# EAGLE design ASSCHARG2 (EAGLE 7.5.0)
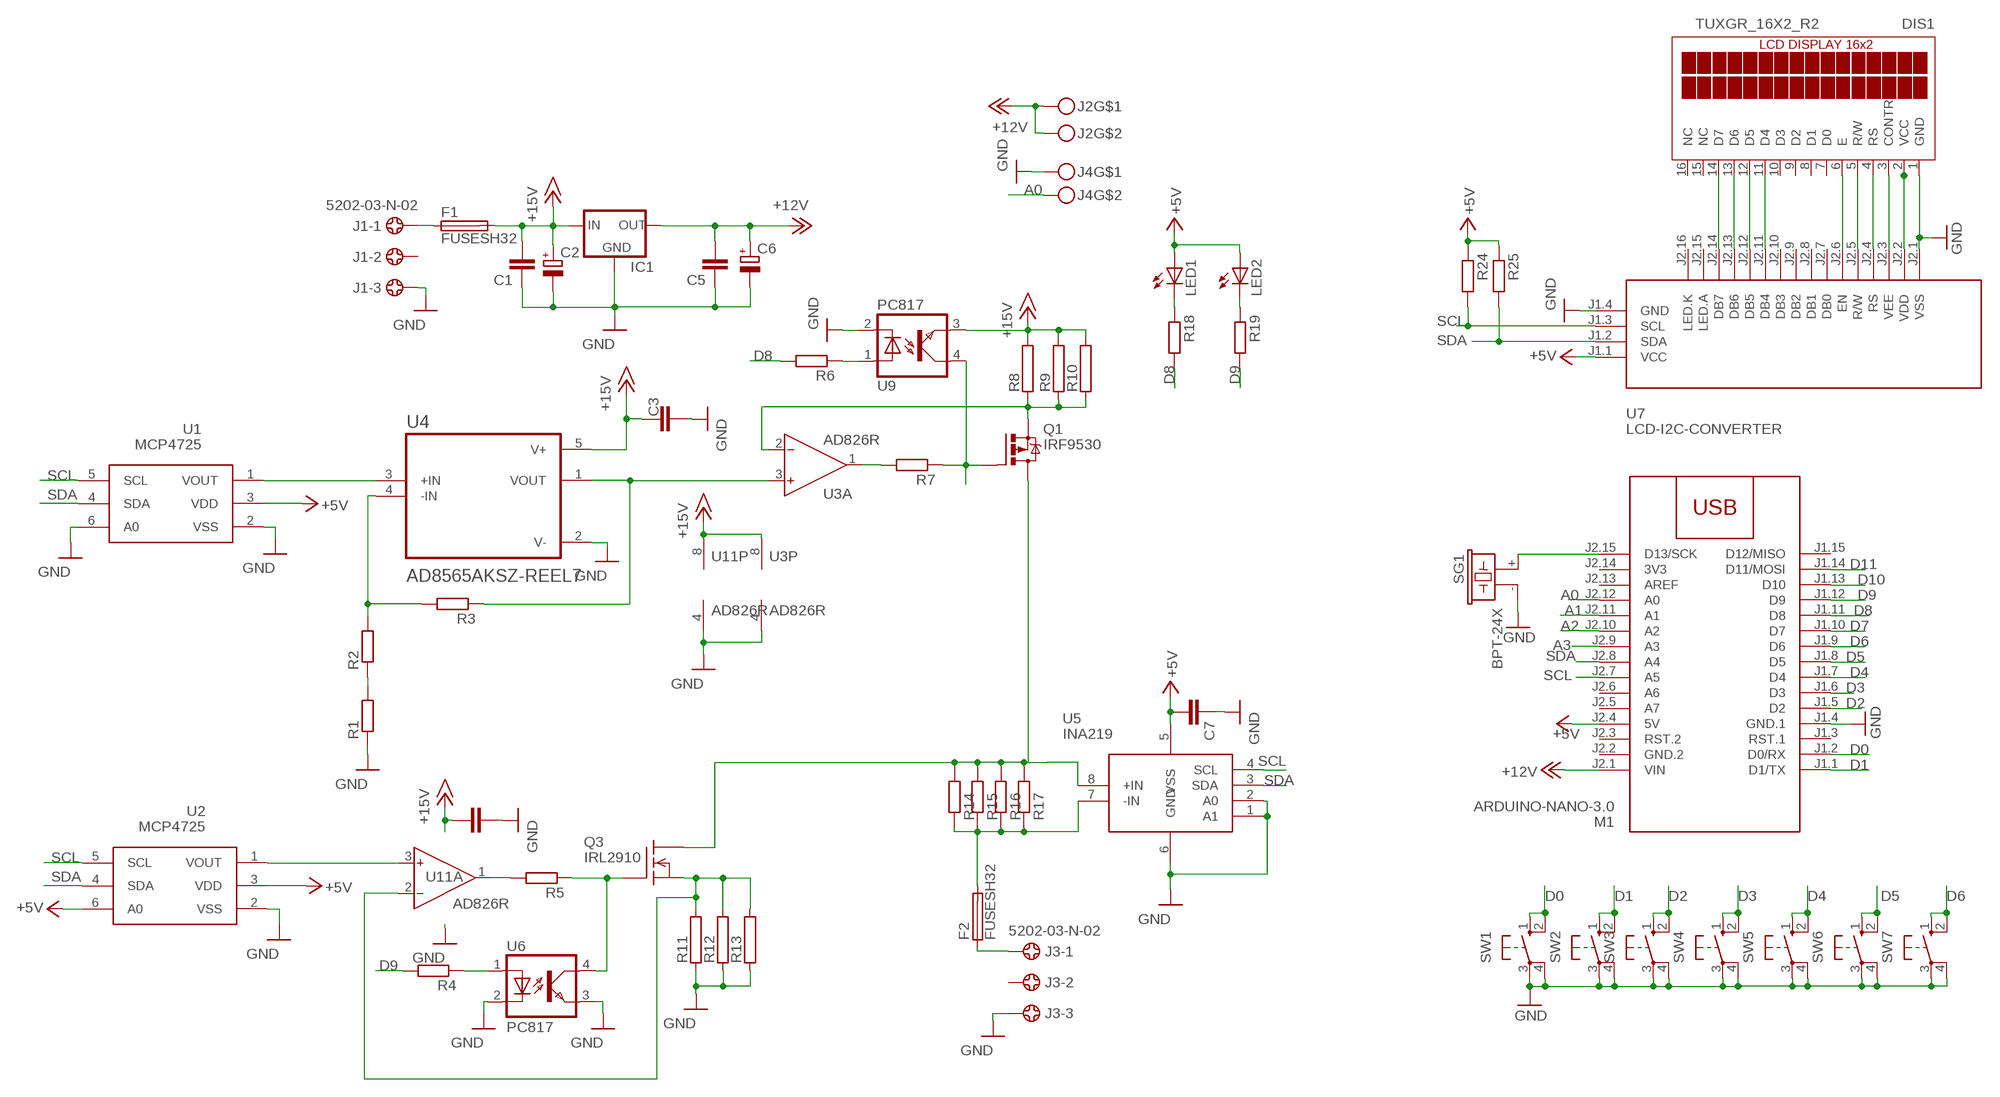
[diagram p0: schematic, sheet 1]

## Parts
C1  C-EUC1206  [C1206]
C2  CPOL-EUE5-10.5  [E5-10,5]
C3  C-EUC1206  [C1206]
C4  C-EUC1206  [C1206]
C5  C-EUC1206  [C1206]
C6  CPOL-EUE2.5-7  [E2,5-7]
C7  C-EUC1206  [C1206]
DIS1  TUXGR_16X2_R2  [TUXGR_16X2_R2]
F1  FUSESH32  [SH32]
F2  FUSESH32  [SH32]
IC1  78XXL  [78XXL]
J1  5202-03-N-02  [5202-03-N-02]
J2  MKDSN1,5-2-5,08  [MKDSN1,5-2-5,08]
J3  5202-03-N-02  [5202-03-N-02]
J4  MKDSN1,5-2-5,08  [MKDSN1,5-2-5,08]
LED1  LED5MM  [LED5MM]
LED2  LED5MM  [LED5MM]
M1  ARDUINO-NANO-3.0  [ARDUINO-NANO-3.0]
Q1  IRF9530  [TO220BV]
Q3  IRL2910  SUP75N06-08  [TO220]
R1  R-EU_R1206  [R1206]
R2  R-EU_R1206  [R1206]
R3  R-EU_R1206  [R1206]
R4  R-EU_R1206  [R1206]
R5  R-EU_R1206  [R1206]
R6  R-EU_R1206  [R1206]
R7  R-EU_R1206  [R1206]
R8  RAC07  [AC07]
R9  RAC07  [AC07]
R10  RAC07  [AC07]
R11  RAC07  [AC07]
R12  RAC07  [AC07]
R13  RAC07  [AC07]
R14  R-EU_R2512  [R2512]
R15  R-EU_R2512  [R2512]
R16  R-EU_R2512  [R2512]
R17  R-EU_R2512  [R2512]
R18  R-EU_R1206  [R1206]
R19  R-EU_R1206  [R1206]
R24  R-EU_R1206  [R1206]
R25  R-EU_R1206  [R1206]
SG1  BPT-24X  [BPT-24X]
SW1  10-XX  [B3F-10XX]
SW2  10-XX  [B3F-10XX]
SW3  10-XX  [B3F-10XX]
SW4  10-XX  [B3F-10XX]
SW5  10-XX  [B3F-10XX]
SW6  10-XX  [B3F-10XX]
SW7  10-XX  [B3F-10XX]
U1  MCP4725  [SOT23-6]
U2  MCP4725  [SOT23-6]
U3  AD826R  [SO8]
U4  AD8565AKSZ-REEL7  [SOT65P210X110-5N]
U5  INA219  [SO08]
U6  PC817  [DIL04]
U7  LCD-I2C-CONVERTER  [LCD-I2C-CONVERTER]
U9  PC817  [DIL04]
U11  AD826R  [SO8]

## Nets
+5V: C7.2 LED1.A LED2.A M1.J2.4(5V) R24.1 R25.1 U1.3(VDD) U2.3(VDD) U2.6(A0) U5.5(VSS) U7.J1.1(VCC)
+12V: C5.2 C6.+ IC1.OUT J2.1 J2.2 M1.J2.1(VIN)
+15V: C1.2 C2.+ C3.1 C4.1 F1.2A IC1.IN R8.2 R9.2 R10.2 U3.8(P:V+) U4.5(V+) U9.3(EMIT) U11.8(P:V+)
A0: J4.2 M1.J2.12(A0)
A1: M1.J2.11(A1)
A2: M1.J2.10(A2)
A3: M1.J2.9(A3)
D0: M1.J1.2(D0/RX) SW1.1(S) SW1.2(S1)
D1: M1.J1.1(D1/TX) SW2.1(S) SW2.2(S1)
D2: M1.J1.5(D2) SW3.1(S) SW3.2(S1)
D3: M1.J1.6(D3) SW4.1(S) SW4.2(S1)
D4: M1.J1.7(D4) SW5.1(S) SW5.2(S1)
D5: M1.J1.8(D5) SW6.1(S) SW6.2(S1)
D6: M1.J1.9(D6) SW7.1(S) SW7.2(S1)
D7: M1.J1.10(D7)
D8: M1.J1.11(D8) R6.2 R18.2
D9: M1.J1.12(D9) R4.2 R19.2
D10: M1.J1.13(D10)
D11: M1.J1.14(D11/MOSI)
GND: C1.1 C2.- C3.2 C4.2 C5.1 C6.- C7.1 DIS1.1(GND) IC1.GND J1.3 J3.3 J4.1 M1.J1.4(GND.1) R1.1 R11.1 R12.1 R13.1 SG1.- SW1.3(P) SW1.4(P1) SW2.3(P) SW2.4(P1) SW3.3(P) SW3.4(P1) SW4.3(P) SW4.4(P1) SW5.3(P) SW5.4(P1) SW6.3(P) SW6.4(P1) SW7.3(P) SW7.4(P1) U1.2(VSS) U1.6(A0) U2.2(VSS) U3.4(P:V-) U4.2(V-) U5.1(A1) U5.2(A0) U5.6(GND) U6.2(C) U6.3(EMIT) U7.J1.4(GND) U7.J2.1(VSS) U9.2(C) U11.4(P:V-)
N$1: DIS1.14(D7) U7.J2.14(DB7)
N$2: DIS1.13(D6) U7.J2.13(DB6)
N$3: DIS1.12(D5) U7.J2.12(DB5)
N$4: DIS1.11(D4) U7.J2.11(DB4)
N$5: DIS1.6(E) U7.J2.6(EN)
N$6: DIS1.5(R/W) U7.J2.5(R/W)
N$7: DIS1.4(RS) U7.J2.4(RS)
N$8: U2.1(VOUT) U11.3(A:IN+)
N$9: R2.2 R3.2 U4.4(-IN)
N$10: DIS1.3(CONTR) U7.J2.3(VEE)
N$11: DIS1.2(VCC) U7.J2.2(VDD)
N$12: R1.2 R2.1
N$13: R3.1 U3.3(A:IN+) U4.1(VOUT)
N$14: U1.1(VOUT) U4.3(+IN)
N$15: R5.2 U11.1(A:OUT)
N$16: Q3.1(G) R5.1 U6.4(COL)
N$17: Q3.3(S) R11.2 R12.2 R13.2 U11.2(A:IN-)
N$18: F2.2A R14.1 R15.1 R16.1 R17.1 U5.7(-IN)
N$19: R4.1 U6.1(A)
N$21: R6.1 U9.1(A)
N$22: Q1.G R7.1 U9.4(COL)
N$23: Q1.D Q3.2(D) R14.2 R15.2 R16.2 R17.2 U5.8(+IN)
N$24: Q1.S R8.1 R9.1 R10.1 U3.2(A:IN-)
N$25: LED1.K(C) R18.1
N$26: R7.2 U3.1(A:OUT)
N$27: LED2.K(C) R19.1
N$28: M1.J2.15(D13/SCK) SG1.+
N$29: F1.1A J1.1
N$30: F2.1A J3.1
SCL: M1.J2.7(A5) R24.2 U1.5(SCL) U2.5(SCL) U5.4(SCL) U7.J1.3(SCL)
SDA: M1.J2.8(A4) R25.2 U1.4(SDA) U2.4(SDA) U5.3(SDA) U7.J1.2(SDA)
Unconnected: DIS1.7(D0) DIS1.8(D1) DIS1.9(D2) DIS1.10(D3) DIS1.15(NC) DIS1.16(NC) J1.2 J3.2 M1.J1.3(RST.1) M1.J1.15(D12/MISO) M1.J2.3(RST.2) M1.J2.5(A7) M1.J2.6(A6) M1.J2.13(AREF) U3.5(B:IN+) U3.6(B:IN-) U3.7(B:OUT) U7.J2.7(DB0) U7.J2.8(DB1) U7.J2.9(DB2) U7.J2.10(DB3) U7.J2.15(LED.A) U7.J2.16(LED.K) U11.5(B:IN+) U11.6(B:IN-) U11.7(B:OUT)

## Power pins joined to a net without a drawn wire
3V3: M1.J2.14(3V3)
GND.2: M1.J2.2(GND.2)

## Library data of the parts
C1 C3-C5 C7 = rcl:C-EU: CAPACITOR, European symbol
C2 C6 = rcl:CPOL-EU: POLARIZED CAPACITOR, European symbol
DIS1 = display-lcd:TUXGR_16X2_R2: Tuxgraphics LCD display 16x2 characters reflective, without background light Source: tuxgr_12x2_r2.pdf; OC_FARNELL: unknown; OC_NEWARK: unknown
F1 F2 = fuse:FUSE: Fuse; OC_FARNELL: unknown; OC_NEWARK: unknown
IC1 = v-reg:78XXL: VOLTAGE REGULATOR
J1 J3 = con-ebyelectro:5202-03-N-02: Barrier Blocks Sreies 5202 Source: http://www.ebyelectro.com/PDF/5202-XX-N-02.pdf; OC_FARNELL: unknown; OC_NEWARK: unknown
J2 J4 = con-phoenix-508:MKDSN1,5-2-5,08
LED1 LED2 = led:LED: LED
M1 = diy-modules:ARDUINO-NANO-3.0: Arduino Nano 3.0 and compatible devices More details available here: https://www.arduino.cc/en/Main/ArduinoBoardNano Click here to find device on ebay.com
Q1 = transistor-power:IRF9530: P-CHANNEL HEXFET POWER-MOS-FET Source: http://www.irf.com/product-info/datasheets/data/irf9530.pdf
Q3 = transistor-fet:SUP75N06-08: N-Channel Enhancement MOSFET 60V; 75A; 0,008Ohm
R1-R7 R14-R19 R24 R25 = rcl:R-EU_: RESISTOR, European symbol
R8-R13 = resistor-power:R: Power Resitor; OC_FARNELL: unknown; OC_NEWARK: unknown
SG1 = buzzer:BPT-24X; OC_FARNELL: unknown; OC_NEWARK: unknown
SW1-SW7 = switch-omron:10-XX: OMRON SWITCH; MPN: B3F-1000; OC_FARNELL: 176432; OC_NEWARK: 36M3542
U1 U2 = linear:MCP4725
U3 U11 = analog-devices:AD826: High-Speed, Low-Power Dual Operational Amplifier Source: http://www.analog.com/static/imported-files/data_sheets/AD826.pdf; MF: ALTERA CORPORATION; MPN: AD826AR; OC_FARNELL: 1651291; OC_NEWARK: 05F7688
U4 = AD8565AKSZ-REEL7:AD8565AKSZ-REEL7: Check availability; AVAILABILITY: In Stock; CHECK_PRICES: https://www.snapeda.com/parts/AD8565AKSZ-REEL7/Analog+Devices/view-part/?ref=eda; DESCRIPTION: Standard (General Purpose) Amplifier 1 Circuit Rail-to-Rail SC-70-5; MF: Analog Devices; MP: AD8565AKSZ-REEL7; PACKAGE: Package; PRICE: None; SNAPEDA_LINK: https://www.snapeda.com/parts/AD8565AKSZ-REEL7/Analog+Devices/view-part/?ref=snap
U5 = burr-brown:INA219: Bidirectional Current/Power Monitor With I2C Interface
U6 U9 = optocoupler:PC817: SHARP OPTO COUPLER; MPN: PC817X4J000F; OC_FARNELL: 9707727; OC_NEWARK: 97K7059
U7 = diy-modules:LCD-I2C-CONVERTER: I2C Bus to 4-Bit Parallel LCD Interface with LED backlight driver

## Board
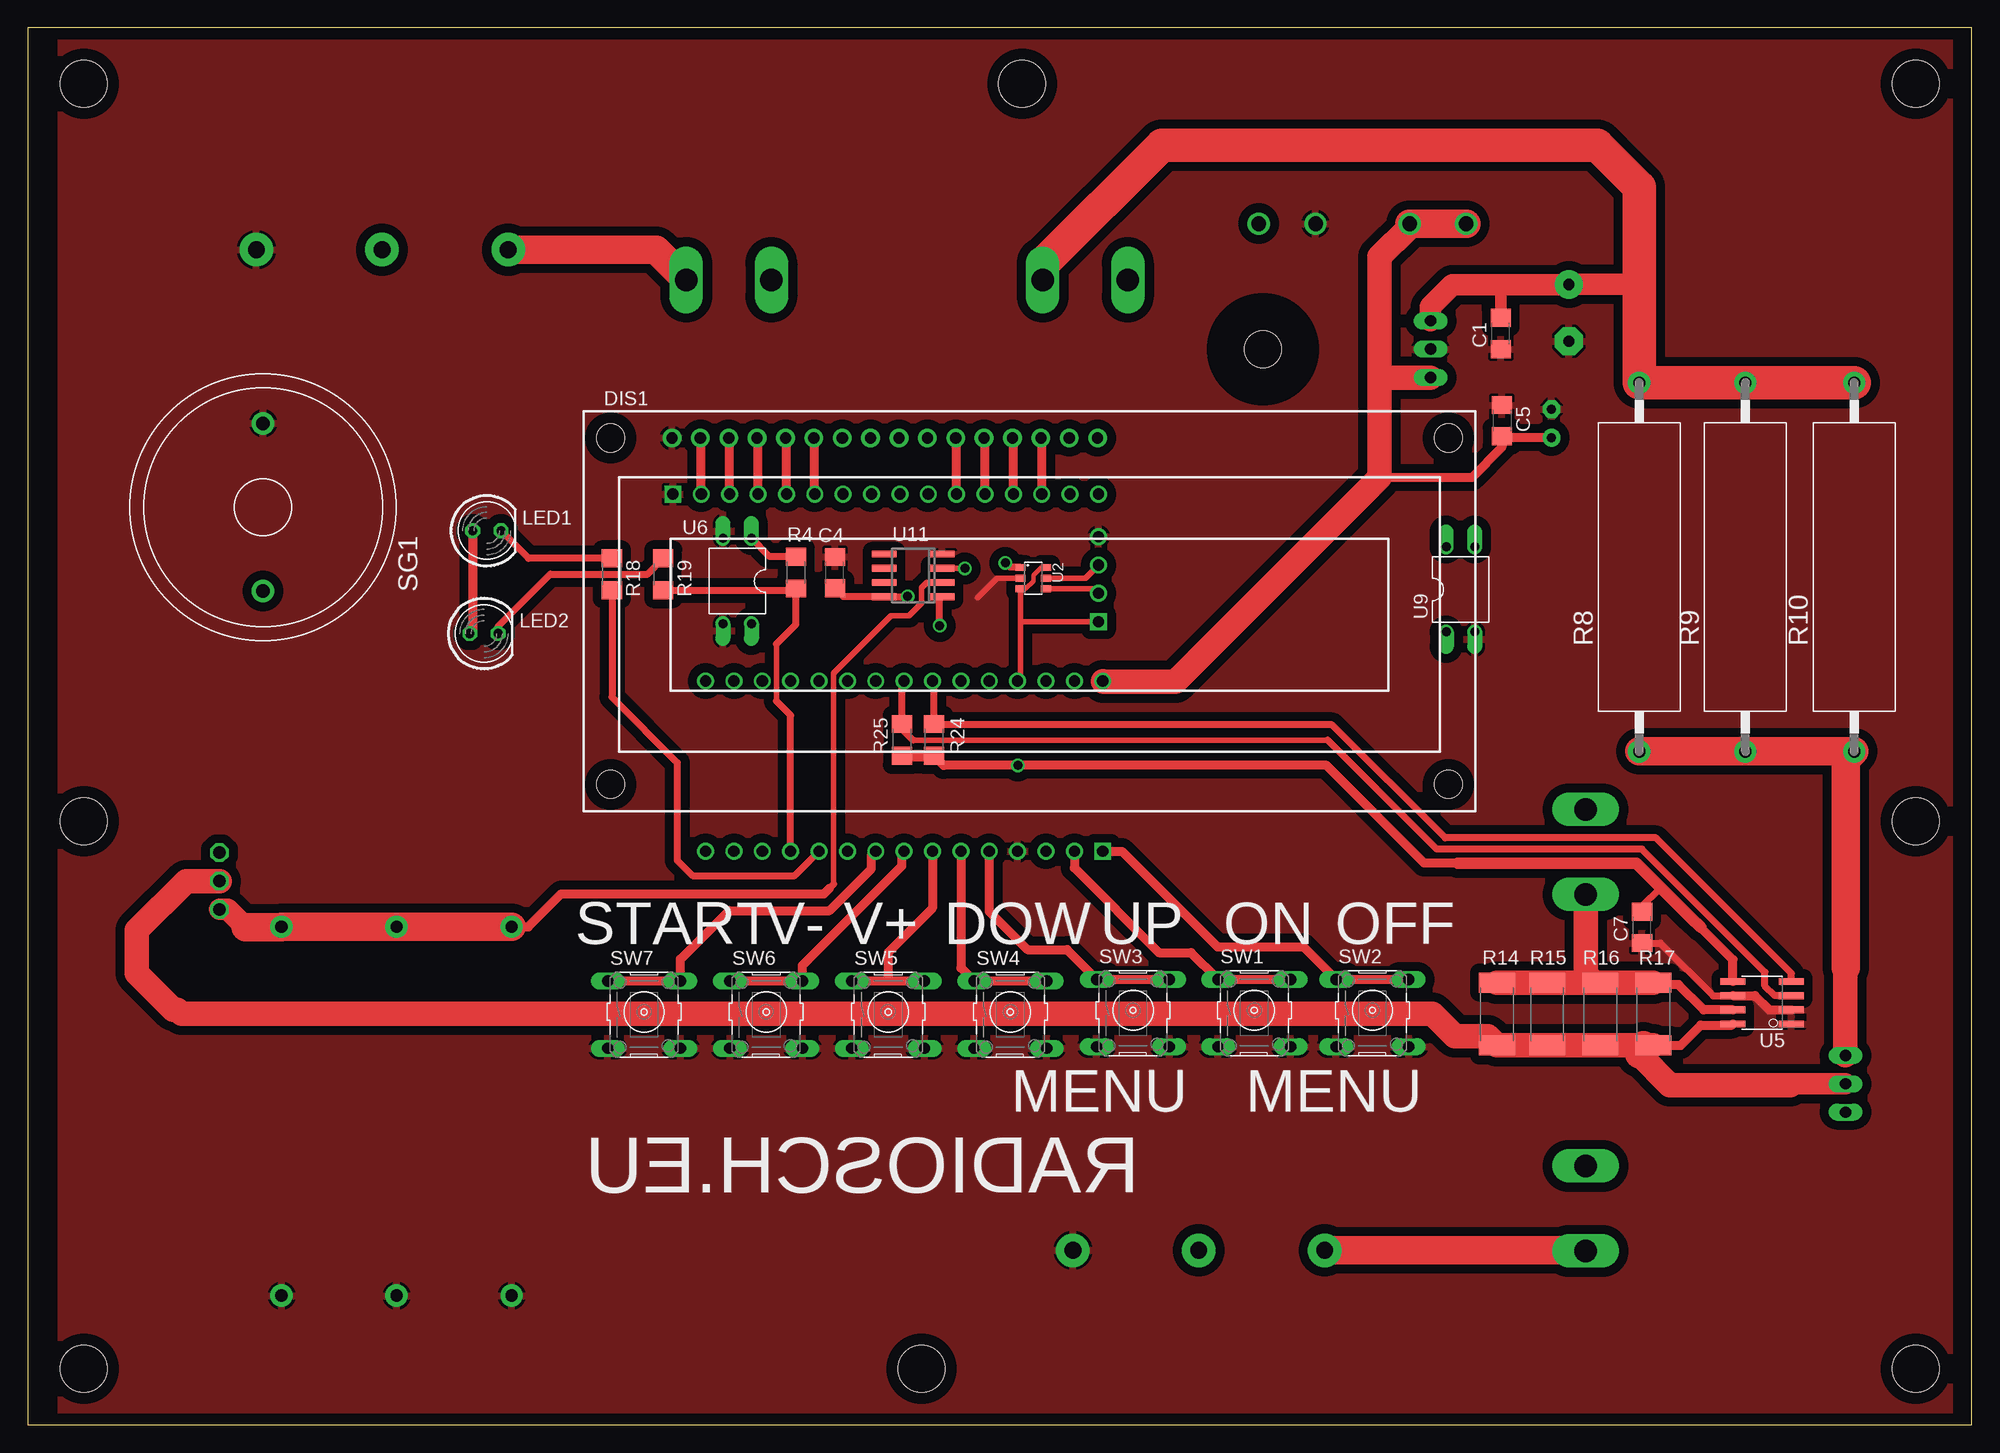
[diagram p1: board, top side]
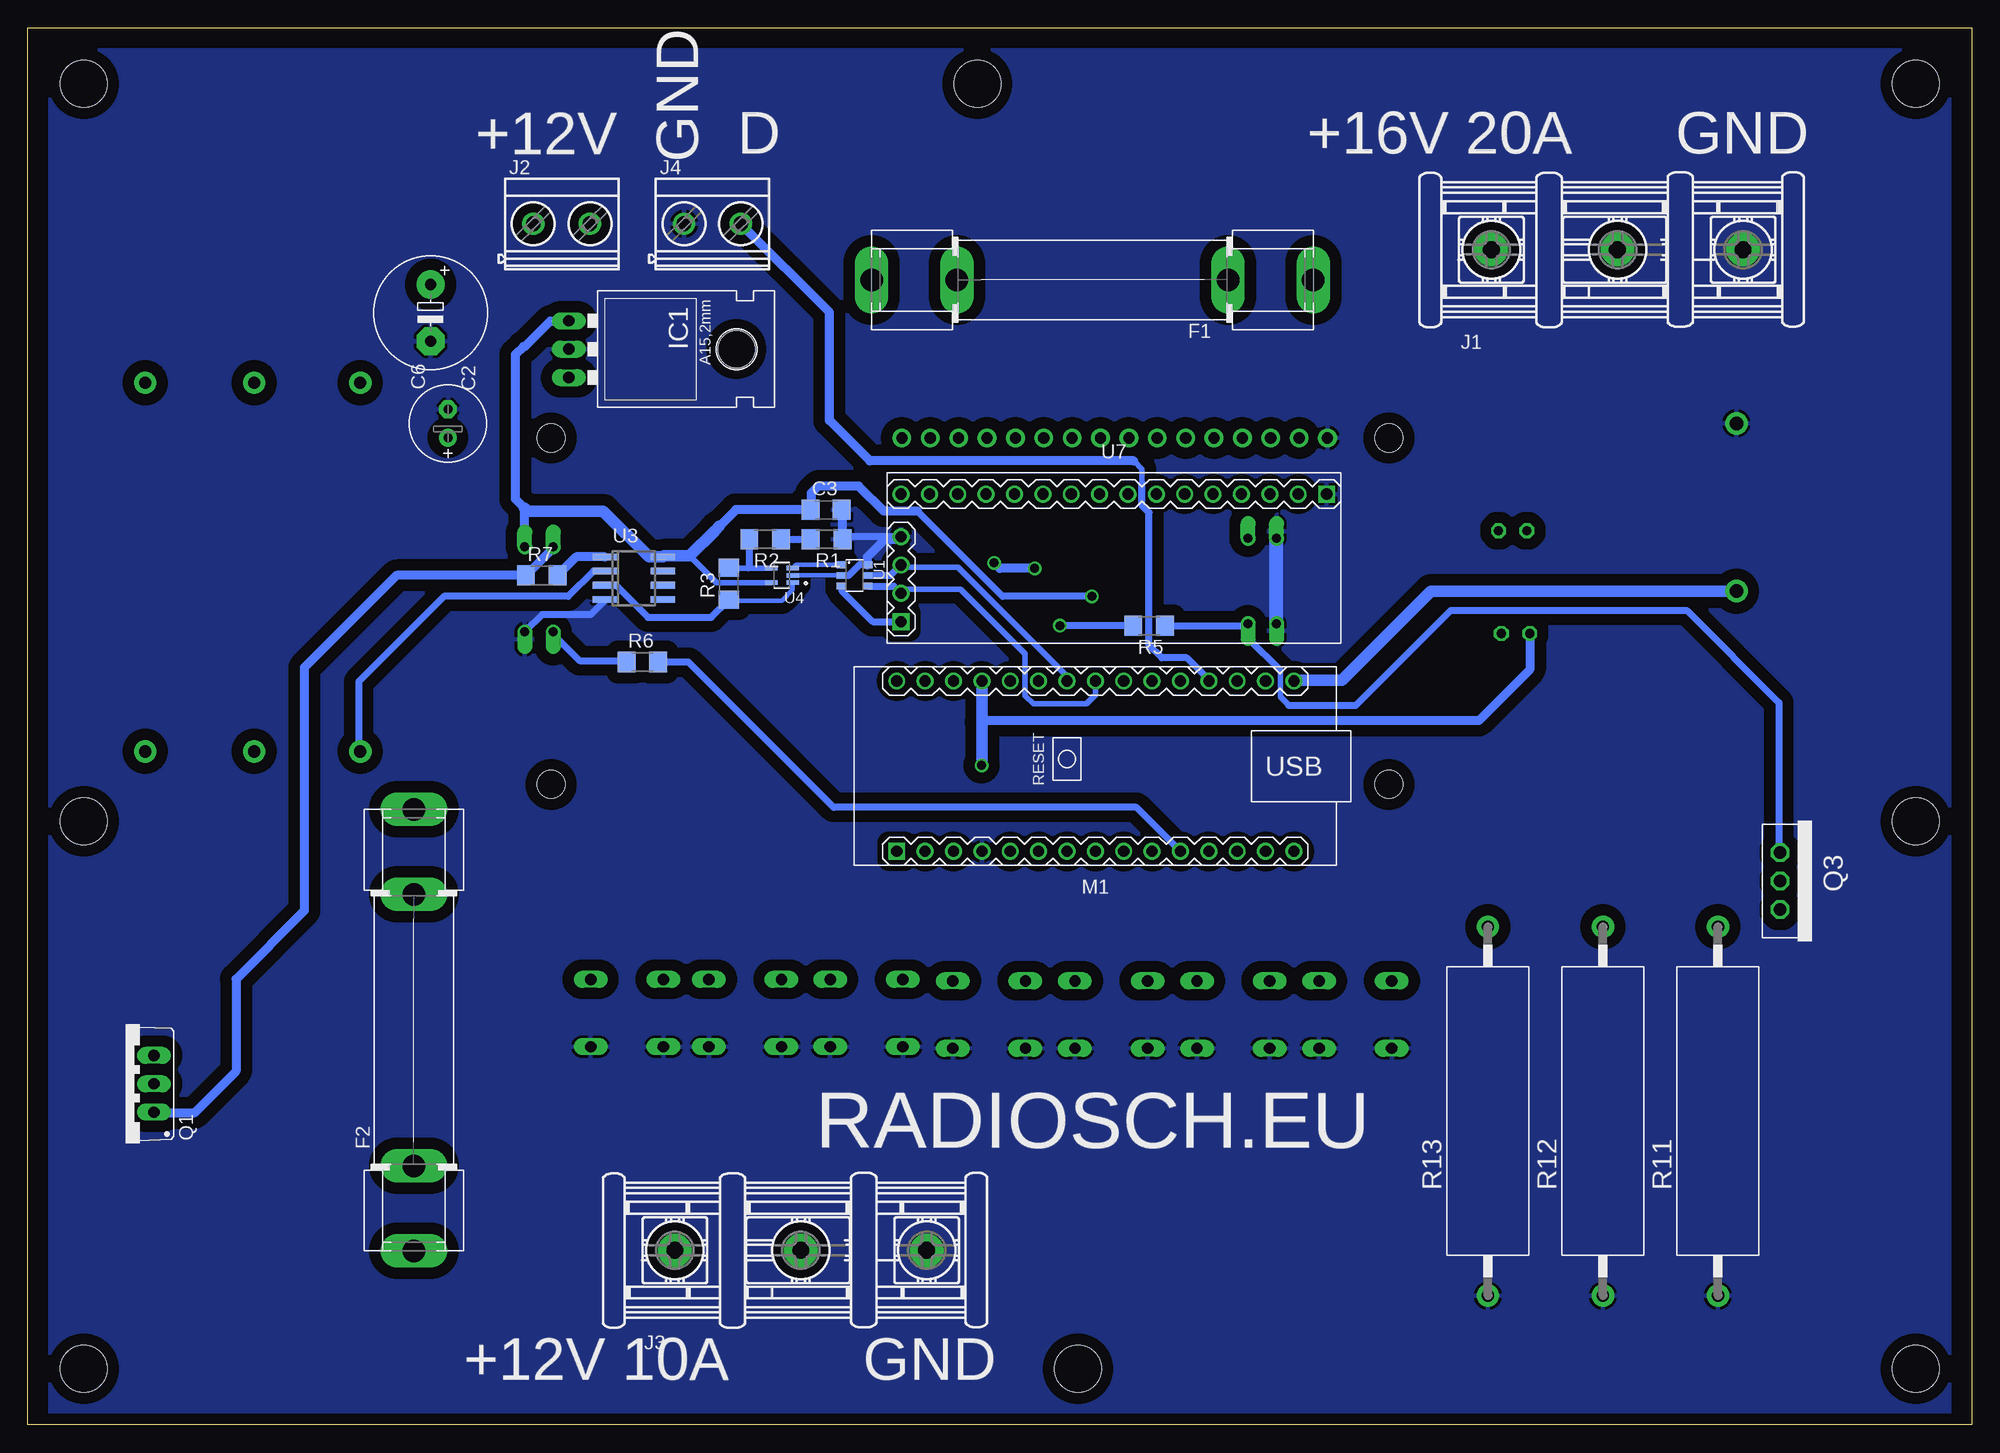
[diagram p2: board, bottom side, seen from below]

Size 174 x 125 mm. Coordinates in mm from the lower left corner, seen from the top.
Outline: 0,0 174,0 174,125 0,125 0,0
Copper layers (1*16): Top 0.035mm / dielectric 1.5mm / Bottom 0.035mm
Design rules "default": minimum track width 10mil, minimum drill 24mil, track to track 8mil, track to pad 8mil, pad to pad 8mil, via to via 8mil, smd to smd 8mil, copper to edge 40mil, drill to drill 8mil, minimum pad ring 10mil, minimum via ring 8mil, stop-mask expansion 4mil, vias tented up to drill 0mil, thermal gap 10mil
Holes 4.2 mm at 5,120 89,120 169,120 5,54 169,54 5,5 80,5 169,5

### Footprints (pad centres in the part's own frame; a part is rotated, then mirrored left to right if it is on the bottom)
C1206 = smd 1.6 x 1.8: 1 -1.4,0; 2 1.4,0
E5-10,5 = drill 1.016 pad 2.54: + -2.54,0 | drill 1.016 pad 2.54 octagon: - 2.54,0
E2,5-7 = drill 0.813 pad 1.6: + -1.27,0 | drill 0.813 pad 1.6 octagon: - 1.27,0
TUXGR_16X2_R2 = drill 1 pad 1.676: 1 -32,15.5; 2 -29.46,15.5; 3 -26.92,15.5; 4 -24.38,15.5; 5 -21.84,15.5; 6 -19.3,15.5; 7 -16.76,15.5; 8 -14.22,15.5; 9 -11.68,15.5; 10 -9.14,15.5; 11 -6.6,15.5; 12 -4.06,15.5; 13 -1.52,15.5; 14 1.02,15.5; 15 3.56,15.5; 16 6.1,15.5 | hole 2.5: -37.5,-15.5; 37.5,-15.5; -37.5,15.5; 37.5,15.5
SH32 = drill 2.007 long: 1A -16.764,0; 1B -9.144,0; 2A 15.144,0; 2B 22.764,0
78XXL = drill 1.016 long: GND 0,-3.81; IN -2.54,-3.81; OUT 2.54,-3.81 | hole 3.302: 0,11.176
5202-03-N-02 = drill 1.5 pad 3: 1 -9.29,0; 2 2,0; 3 13.25,0
MKDSN1,5-2-5,08 = drill 1.3 pad 2: 1 -2.561,0.025; 2 2.519,0.025
LED5MM = drill 0.813 octagon: A -1.27,0; K 1.27,0
ARDUINO-NANO-3.0 = drill 1 square: J1.1 17.78,7.62 | drill 1: J1.2 15.24,7.62; J1.3 12.7,7.62; J1.4 10.16,7.62; J1.5 7.62,7.62; J1.6 5.08,7.62; J1.7 2.54,7.62; J1.8 0,7.62; J1.9 -2.54,7.62; J1.10 -5.08,7.62; J1.11 -7.62,7.62; J1.12 -10.16,7.62; J1.13 -12.7,7.62; J1.14 -15.24,7.62; J1.15 -17.78,7.62; J2.1 17.78,-7.62; J2.2 15.24,-7.62; J2.3 12.7,-7.62; J2.4 10.16,-7.62; J2.5 7.62,-7.62; J2.6 5.08,-7.62; J2.7 2.54,-7.62; J2.8 0,-7.62; J2.9 -2.54,-7.62; J2.10 -5.08,-7.62; J2.11 -7.62,-7.62; J2.12 -10.16,-7.62; J2.13 -12.7,-7.62; J2.14 -15.24,-7.62; J2.15 -17.78,-7.62
TO220BV = drill 1.016 long: D 0,-2.54; G -2.54,-2.54; S 2.54,-2.54
TO220 = drill 1.118 octagon: 1 -2.54,0; 2 0,0; 3 2.54,0
R1206 = smd 1.6 x 1.803: 1 -1.422,0; 2 1.422,0
AC07 = drill 1.1 pad 2: 1 -16.5,0; 2 16.5,0
R2512 = smd 1.8 x 3.2: 1 -2.8,0; 2 2.8,0
BPT-24X = drill 1.2 pad 2: + 7.5,0; - -7.5,0
B3F-10XX = drill 1.016 long: 1 -3.251,2.761; 2 3.251,2.761; 3 -3.251,-3.261; 4 3.251,-3.261
SOT23-6 = smd 0.6 x 0.9: 1 -0.95,-1.15; 2 0,-1.15; 3 0.95,-1.15; 4 0.95,1.15; 5 0,1.15; 6 -0.95,1.15
SO8 = smd 0.6 x 2.2: 1 -1.905,-2.6; 2 -0.635,-2.6; 3 0.635,-2.6; 4 1.905,-2.6; 5 1.905,2.6; 6 0.635,2.6; 7 -0.635,2.6; 8 -1.905,2.6
SOT65P210X110-5N = smd 1.19 x 0.4: 1 -0.96,0.65; 2 -0.96,0; 3 -0.96,-0.65; 4 0.96,-0.65; 5 0.96,0.65
SO08 = smd 0.61 x 2.21: 1 -1.905,-2.616; 2 -0.635,-2.616; 3 0.635,-2.616; 4 1.905,-2.616; 5 1.905,2.616; 6 0.635,2.616; 7 -0.635,2.616; 8 -1.905,2.616
DIL04 = drill 0.813 offset: 1 -1.27,-3.81; 2 1.27,-3.81; 3 1.27,3.81; 4 -1.27,3.81
LCD-I2C-CONVERTER = drill 1 square: J1.1 -19.05,-5.08; J2.1 19.05,6.35 | drill 1: J1.2 -19.05,-2.54; J1.3 -19.05,0; J1.4 -19.05,2.54; J2.2 16.51,6.35; J2.3 13.97,6.35; J2.4 11.43,6.35; J2.5 8.89,6.35; J2.6 6.35,6.35; J2.7 3.81,6.35; J2.8 1.27,6.35; J2.9 -1.27,6.35; J2.10 -3.81,6.35; J2.11 -6.35,6.35; J2.12 -8.89,6.35; J2.13 -11.43,6.35; J2.14 -13.97,6.35; J2.15 -16.51,6.35; J2.16 -19.05,6.35

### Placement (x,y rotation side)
C1  131.85,97.65 90 top
C2  137.95,99.5 270 bottom
C3  102.55,81.88 0 bottom
C4  72.25,76.25 90 top
C5  131.95,89.85 270 top
C6  136.4,89.6 90 bottom
C7  144.5,44.5 90 top
DIS1  89.66,72.8 0 top
F1  75.7,102.45 180 bottom
F2  139.45,32.3 90 bottom
IC1  121.75,96.25 270 bottom
J1  33.7,105.15 0 bottom
J2  126.2,107.45 0 bottom
J3  106.8,15.6 0 bottom
J4  112.7,107.45 0 bottom
LED1  41.08,80 0 top
LED2  40.83,70.8 0 top
M1  78.44,58.93 180 bottom
Q1  165.25,30.5 90 bottom
Q3  17.15,48.65 270 bottom
R1  102.5,79.25 180 bottom
R2  108,79.25 180 bottom
R3  111.25,75.25 90 bottom
R4  68.75,76.25 270 top
R5  73.62,71.5 180 bottom
R6  119,68.25 0 bottom
R7  128,76 0 bottom
R8  144.25,76.75 90 top
R9  153.75,76.75 90 top
R10  163.5,76.75 90 top
R11  22.7,28.05 90 bottom
R12  33,28.05 90 bottom
R13  43.3,28.05 90 bottom
R14  131.5,36.75 270 top
R15  136,36.75 270 top
R16  140.75,36.75 270 top
R17  145.5,36.75 270 top
R18  52.27,76.1 270 top
R19  56.88,76.1 270 top
R24  81.12,61.27 90 top
R25  78.25,61.27 90 top
SG1  21.05,82.1 270 top
SW1  109.79,37.08 0 top
SW2  120.36,37.08 0 top
SW3  98.93,37.08 0 top
SW4  87.95,36.94 0 top
SW5  77.02,36.94 0 top
SW6  66.09,36.94 0 top
SW7  55.16,36.94 0 top
U1  100,76 270 bottom
U2  90,75.75 270 top
U3  119.75,75.75 270 bottom
U4  106.5,76 180 bottom
U5  155.25,37.75 90 top
U6  63.5,75.5 180 top
U7  76.79,76.93 0 bottom
U9  128.25,74.75 0 top
U11  79.25,76 90 top

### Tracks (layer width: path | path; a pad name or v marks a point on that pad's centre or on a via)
+5V  (via drill 0.8)
  Top 0.406: U2.3 89.3,74.8 90,75.5 90,76 90.75,76.75 91.1,76.75 U2.6
  Top 0.5: U2.3 88.85,71.75 | 88.85,71.75 88.85,66.8 M1.J2.4 | U7.J1.1 88.95,71.85 88.85,71.75
  Top 0.61: C7.2 144.5,46.38 146.19,48.06
  Top 0.813: U5.5 152.63,41.62 148.88,45.38 | 128,50.25 125,50.25 116.25,59 v88.62,59 81.98,59 R24.1 | LED1.A 39.8,71.05 LED2.A
  Top 1.016: 128,50.25 144,50.25 146.19,48.06 148.88,45.38 149.75,44.5 | R24.1 R25.1
  Bottom 0.61: U1.3 101.15,74.65 98.38,71.88 95.86,71.88 U7.J1.1
  Bottom 0.813: LED2.A 39.55,67.57 44.12,63 88.47,63 88.6,62.88
  Bottom 1.016: M1.J2.4 88.6,62.88 88.6,59.02 v88.62,59
+12V
  Top 0.813: 121,84.75 129.25,84.75 131.95,87.45 C5.2 132.07,88.33 C6.+
  Top 2.184: J2.2 123.68,107.18 121,104.5 121,93.5 | 121,93.5 121,84.75 102.75,66.5 96.27,66.5 M1.J2.1 | IC1.OUT 121.21,93.71 121,93.5
  Top 2.54: J2.2 J2.1
+15V  (via drill 0.8)
  Top 0.61: v78.75,74.12 78.72,74.09 U11.8 73,74.09 C4.1
  Top 1.016: C1.2 131.85,101.4 131.25,102
  Top 1.93: IC1.IN 125.56,100.06 127.5,102 131.25,102 137.91,102 C2.+ 144.21,102.04 144.25,102
  Top 3: F1.2A 90.84,103.84 101.5,114.5 140.5,114.5 144.25,110.75 144.25,102 R8.2 R9.2 R10.2
  Bottom 0.5: U4.5 112.35,75.35 114.75,77.75
  Bottom 0.61: v78.75,74.12 86.75,74.12 94.38,81.75
  Bottom 0.813: U9.3 129.52,82 130.38,82.86 130.38,95.75 129.65,96.48 129.52,96.48 127.25,98.75 125.6,98.75 IC1.IN | 112.5,80 110.62,81.88 C3.1 103.88,81.95 103.88,83.38 103.25,84 99.62,84 97.38,81.75 94.38,81.75
  Bottom 1.016: 112.12,80.38 112.5,80 114.75,77.75 117.06,77.75 U3.8 118.41,77.66 122.5,81.75 129.27,81.75 129.52,82
A0
  Bottom 0.5: 74.25,84.25 74.25,85.5 75,86.25
  Bottom 0.61: 74.25,84.25 74.25,82.25 73.62,81.62 73.62,69.75 72.5,68.62 70.25,68.62 68.28,66.66 M1.J2.12
  Bottom 0.813: 75,86.25 98.62,86.25 102.25,89.88 102.25,99.54 J4.2
D0
  Top 0.813: M1.J1.2 93.68,49.82 101.25,42.25 104.13,42.25 SW1.1 SW1.2
D1
  Top 0.813: SW2.2 SW2.1 114.2,42.75 106.5,42.75 97.94,51.31 M1.J1.1
D2
  Top 0.813: M1.J1.5 86.06,45.94 89.5,42.5 93.02,42.5 SW3.1 SW3.2
D3
  Top 0.813: M1.J1.6 83.52,40.88 SW4.1 SW4.2
D4
  Top 0.813: SW5.1 76.75,39.7 | 76.75,39.7 SW5.2 | M1.J1.7 80.98,46.23 77,42.25 77,39.95 76.75,39.7
D5
  Top 0.813: SW6.1 SW6.2 69.34,41.09 78.25,50 78.25,51.12 M1.J1.8
D6
  Top 0.813: SW7.1 SW7.2 58.41,41.66 62.75,46 71.75,46 75.5,49.75 75.5,50.91 M1.J1.9
D8
  Top 0.61: R18.2 52.27,65.1 58.12,59.25 58.12,50.5 59.5,49.12 68.64,49.12 M1.J1.11
  Bottom 0.61: M1.J1.11 74.75,55.25 101.88,55.25 114.88,68.25 R6.2
D9
  Top 0.5: 67,64.75 67,69.88
  Top 0.61: M1.J1.12 68.28,63.47 67,64.75 | 67,69.88 68.75,71.62 R4.2 68.6,74.68 R19.2
GND
  Top 0.5: U2.2 86.75,75.75 85,74
  Top 0.61: C7.1 146.15,43.1 150.88,38.38 U5.6
  Top 0.813: U5.6 154.62,38.38 155.88,37.12 157.86,37.12 U5.2
  Bottom 0.406: U4.2 U1.2
  Bottom 0.61: U1.2 100.5,76 99.5,77 98.9,77 U1.6 | U3.4 122.35,73.78 123.62,72.5 127.96,72.5 U9.2 | U7.J1.4 100.86,79.47 R1.1
  Bottom 0.813: U1.6 98.85,77.65 97.25,79.25 96.06,79.25 U7.J1.4 | R1.1 101.08,81.81 C3.2
  Bottom 1.27: U6.3 U6.2
  pour Top (isolate 0.813): 3,124 172,124 172,1 3,1
  pour Bottom (isolate 1.016): 2,123 172,123 172,1 2,1
N$1
  Top 0.813: U7.J2.14 90.76,88.22 DIS1.14
N$2
  Top 0.813: U7.J2.13 88.22,88.22 DIS1.13
N$3
  Top 0.813: U7.J2.12 85.68,88.22 DIS1.12
N$4
  Top 0.813: U7.J2.11 83.14,88.22 DIS1.11
N$5
  Top 0.813: U7.J2.6 70.44,88.22 DIS1.6
N$6
  Top 0.813: U7.J2.5 67.9,88.22 DIS1.5
N$7
  Top 0.813: U7.J2.4 65.36,88.22 DIS1.4
N$8  (via drill 0.8)
  Top 0.5: U11.3 83.61,76.64 v83.88,76.62 | 88.8,76.75 U2.1
  Top 0.61: 88.8,76.75 87.88,76.75 v87.5,77.12
  Bottom 0.813: v83.88,76.62 87,76.62 v87.5,77.12
N$9
  Bottom 0.5: U4.4 109.5,76.65 111.23,76.65 R3.2
  Bottom 0.61: R2.2 109.42,76.73 109.5,76.65
N$10
  Top 0.813: U7.J2.3 62.82,88.22 DIS1.3
N$11
  Top 0.813: U7.J2.2 60.28,88.22 DIS1.2
N$12
  Bottom 0.61: R2.1 R1.2
N$13
  Bottom 0.406: U4.1 105.54,74.71 106.5,73.75 111.17,73.75 R3.1
  Bottom 0.61: U3.3 121.36,75.11 118.5,72.25 112.83,72.25 R3.1
N$14
  Bottom 0.406: U1.1 105.24,76.95 U4.3
N$15  (via drill 0.8)
  Top 0.61: v81.62,71.5 81.62,73.87 U11.1
  Bottom 0.61: R5.2 v81.62,71.5
N$16
  Bottom 0.5: 61.88,67.5 61.88,65.12 61.12,64.38
  Bottom 0.61: 61.88,67.5 64.77,70.39 U6.4 64.96,71.5 R5.1 | 61.12,64.38 55.12,64.38 46.62,72.88 25.5,72.88 17.25,64.62 17.25,51.29 Q3.1
N$17
  Top 0.5: 72.12,48.38 72.12,67.25 77.25,72.38 78.88,72.38 80,73.5 80,74.88 80.5,75.38 81.84,75.38 U11.2
  Top 0.61: 71.75,48 72.12,48.38
  Top 0.813: R13.2 44.8,44.55 47.75,47.5 71.25,47.5 71.75,48
  Top 1.93: Q3.3 17.89,46.11 19.5,44.5
  Top 2.54: 19.5,44.5 22.65,44.5 R11.2 R12.2 R13.2
N$18
  Top 0.813: U5.7 150.01,37.12 147.75,39.38 145.68,39.38 R17.1
  Top 2.184: R14.1 R15.1 140.25,39.55 | 140.25,39.55 R16.1 R17.1 | F2.2A 139.45,40.35 140.25,39.55
N$19
  Top 0.61: R4.1 66.41,77.67 U6.1
N$21
  Bottom 0.61: U9.1 126.98,70.73 124.62,68.38 120.55,68.38 R6.1
N$22
  Bottom 0.813: U9.4 126.98,78.44 R7.1 141,76 149.25,67.75 149.25,46 155.38,39.88 155.38,31.62 159.12,27.88 162.62,27.88 Q1.G
N$23
  Top 0.813: R17.2 147.95,33.95 149.75,35.75 152.54,35.75 U5.8
  Top 1.93: Q1.D 157.88,30.5 157.75,30.38
  Top 2.184: Q3.2 14.15,48.65 9.75,44.25 9.75,40.38 13,37.12 13.38,37.12 13.75,36.75 125.75,36.75 127.75,34.75 130.7,34.75 R14.2 R15.2 R16.2 144.62,33.95 R17.2 | 157.75,30.38 147,30.38 144.25,33.12
  Top 2.54: 144.25,33.12 144.25,33.58 144.62,33.95
N$24
  Top 2.184: Q1.S 162.71,40.84 162.75,40.88
  Top 2.54: R8.1 R9.1 R10.1 162.75,59.5 162.75,40.88
  Bottom 0.61: U3.2 123.36,76.39 125.62,74.12 136.75,74.12 144.38,66.5 144.38,60.38 R8.1
N$25
  Top 0.61: R18.1 44.82,77.52 LED1.K
N$26
  Bottom 0.813: U3.1 124.92,77.66 R7.2
N$27
  Top 0.61: LED2.K 42.09,71.47 46.75,76.12 55.48,76.12 R19.1
N$28
  Bottom 1.016: SG1.+ 48.4,74.6 56.38,66.62 60.59,66.62 M1.J2.15
N$29
  Top 2.54: J1.1 56.24,105.15 F1.1A
N$30
  Top 2.54: J3.1 139.39,15.6 F2.1A
SCL
  Top 0.5: U2.5 94.66,75.75 U7.J1.3
  Top 0.61: R24.2 81.12,63.25 | 81.12,63.25 81.12,66.41 M1.J2.7 | U5.4 157.87,40.38 145.75,52.5 126.88,52.5 116.75,62.62 81.75,62.62 81.12,63.25
  Bottom 0.5: M1.J2.7 80.98,66.98 90.75,76.75 95.66,76.75 U7.J1.3
  Bottom 0.61: U1.5 96.77,76 U7.J1.3
SDA
  Top 0.5: U2.4 95.43,74.8 U7.J1.2 | 116.38,61.25 79.25,61.25
  Top 0.61: U5.3 156.37,38.38 155.5,39.25 155.5,40.5 144.5,51.5 126.12,51.5 116.38,61.25 | 95.95,74.5 U7.J1.2 | 79.25,61.25 78.25,62.25 R25.2 78.25,66.36 M1.J2.8
  Bottom 0.5: M1.J2.8 78.44,65.31 79.25,64.5 84,64.5 84.75,65.25 84.75,69 90.5,74.75 95.48,74.75 U7.J1.2
  Bottom 0.61: U1.4 96.5,75.05 U7.J1.2

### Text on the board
tPlace: START | V- | V+ | DOW | UP | ON | OFF | MENU | MENU | RADIOSCH.EU
bPlace: +12V | GND | +16V 20A | D | GND | RADIOSCH.EU | GND | +12V 10A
